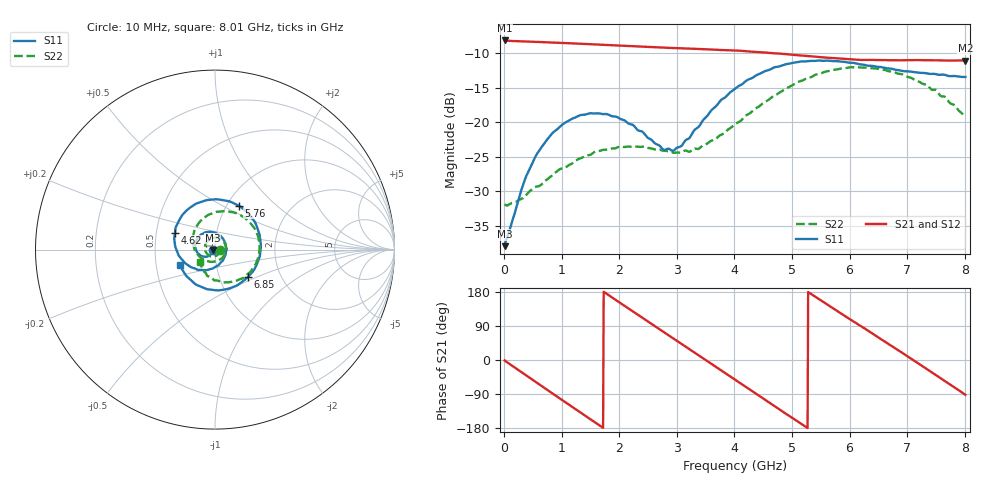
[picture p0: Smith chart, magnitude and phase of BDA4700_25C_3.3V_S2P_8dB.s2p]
!Agilent Technologies,E5071B,MY42404982,A.09.10
!Date: Mon Oct 20 18:06:21 2025
!Data & Calibration Information:
!Freq	S11:SOLT2(ON)	S21:SOLT2(ON)	S12:SOLT2(ON)	S22:SOLT2(ON)
# Hz S RI R 50
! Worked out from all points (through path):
!   801 points, 10 MHz to 8.01 GHz, reference 50 ohm
!   highest |S21| = -8.12 dB at 10 MHz (marker M1); lowest = -11.1 dB at 8.01 GHz (marker M2)
!   group delay of S21, straight-line fit = 281 ps
!   lowest |S11| = -38.0 dB at 10 MHz (marker M3), VSWR 1.03, Z = 48.8 - j0.169 ohm
!   |S11| at or under -10 dB: start of sweep to end of sweep
!   |S22| runs from -32.1 to -12.0 dB; largest |S21 - S12| = 0.0044
!   S11 on the Smith chart (normalised r, x): 10 MHz: 0.98, -0.00; 4.62 GHz: 0.63, +0.12; 5.76 GHz: 1.13, +0.60; 6.85 GHz: 1.37, -0.44; 8.01 GHz: 0.67, -0.12
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1e7  -0.0125 -0.00173  0.3926 -0.00845  0.3924 -0.00892  0.0254 -0.00134
3.5e8  -0.0244 -0.0279  0.3083 -0.2329  0.3078 -0.2331  0.0205 -0.0199
5.7e8  -0.0439 -0.039  0.1914 -0.3321  0.1911 -0.3321  0.0106 -0.0325
9.5e8  -0.0868 -0.0275  -0.0626 -0.3723  -0.0625 -0.3727  -0.0253 -0.0374
1.35e9  -0.1108 0.0227  -0.2882 -0.234  -0.2879 -0.2343  -0.0551 -0.00294
1.64e9  -0.0952 0.0667  -0.3618 -0.0586  -0.3619 -0.0587  -0.0518 0.0337
1.93e9  -0.0549 0.0954  -0.3384 0.1269  -0.3385 0.127  -0.0218 0.0608
2.32e9  0.0125 0.087  -0.1761 0.3081  -0.176 0.3082  0.0314 0.0587
2.68e9  0.057 0.0378  0.0415 0.3474  0.0409 0.3472  0.0611 0.0155
2.95e9  0.0602 -0.017  0.1943 0.2864  0.1936 0.2861  0.0555 -0.0232
3.37e9  0.0104 -0.0915  0.3314 0.0787  0.3318 0.0786  0.00894 -0.0633
3.68e9  -0.0644 -0.1138  0.3196 -0.1043  0.3197 -0.1054  -0.0411 -0.0637
4.01e9  -0.1524 -0.0858  0.2053 -0.2607  0.2057 -0.2602  -0.0902 -0.0347
4.62e9  -0.223 0.0931  -0.1295 -0.2912  -0.1291 -0.2915  -0.1188 0.0889
5e9  -0.1592 0.2169  -0.2738 -0.1432  -0.2745 -0.144  -0.0648 0.1738
5.35e9  -0.0346 0.277  -0.2981 0.04  -0.2984 0.0382  0.033 0.212
5.76e9  0.1315 0.245  -0.1946 0.2171  -0.1941 0.2173  0.1625 0.1787
6.2e9  0.2428 0.1008  0.00461 0.2836  0.00823 0.2844  0.2447 0.0508
6.68e9  0.2264 -0.0957  0.2103 0.1879  0.2109 0.1876  0.2106 -0.1038
6.85e9  0.1839 -0.1527  0.2549 0.1195  0.2556 0.118  0.1731 -0.1439
7.37e9  -0.00756 -0.2253  0.252 -0.1275  0.2521 -0.1276  0.031 -0.1801
8.01e9  -0.1946 -0.0877  -0.00879 -0.2801  -0.00763 -0.2803  -0.086 -0.0679
